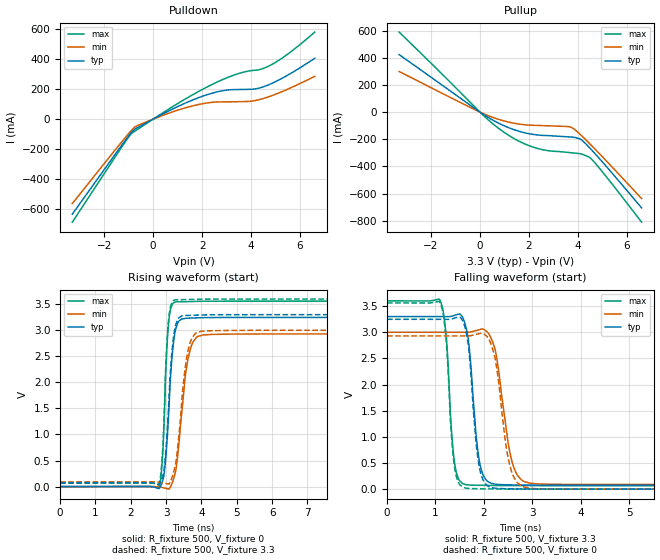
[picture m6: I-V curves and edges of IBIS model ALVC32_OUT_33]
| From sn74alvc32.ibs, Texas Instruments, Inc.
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[Model]   ALVC32_OUT_33
Model_type  Output
Vref =   0
Rref =   500
Cref =   50p
Vmeas =   1.5
| variable   typ   min   max
C_comp   7.48pF   5.11pF   11.40pF
| C_pullup   8.30pF   5.11pF   11.40pF
| C_pulldown   6.66pF   5.16pF   9.51pF
[Temperature Range]   40   100   -40
| Ambient temperature   25   85   -40
[Voltage range]   3.3   3   3.6
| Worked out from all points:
|   slope of the pulldown table from 0 to 0.495 V, typ, clamps not added: 11.6 ohm
|   slope of the pullup table from 0 to 0.495 V, typ, clamps not added: 8.84 ohm
|   rising waveform, R_fixture 500, V_fixture 0: 20-80 % time 181ps typ, 265ps min, 127ps max; typ from 0 V to 3.25 V
|   falling waveform, R_fixture 500, V_fixture 3.3: 20-80 % time 175ps typ, 264ps min, 136ps max; typ from 3.3 V to 0.073 V
|   rising waveform, R_fixture 500, V_fixture 3.3: 20-80 % time 179ps typ, 255ps min, 126ps max; typ from 0.073 V to 3.3 V
|   falling waveform, R_fixture 500, V_fixture 0: 20-80 % time 172ps typ, 243ps min, 137ps max; typ from 3.25 V to 0 V
[Pulldown]
| ALVC32_OUT_33
|   Voltage   I(typ)   I(min)   I(max)
-3.3V     -631.7mA   -561.5mA   -685mA
-1.115V   -136.4mA   -118.3mA   -145.6mA
-910mV    -93.12mA   -79.48mA   -100.6mA
-740mV    -66.58mA   -52.27mA   -79.35mA
825mV     69.55mA    49.91mA    85.75mA
2.12V     157.8mA    105.3mA    206.7mA
2.98V     192.3mA    114.9mA    272.7mA
3.985V    198.5mA    119.1mA    321.9mA
4.4V      209.9mA    132.7mA    331.5mA
4.855V    238mA      156.6mA    363.9mA
5.605V    302.5mA    207mA      445.3mA
6.6V      404.7mA    284.5mA    578.6mA
[Pullup]
| ALVC32_OUT_33
|   Voltage   I(typ)   I(min)   I(max)
-3.3V     423.4mA    299.2mA    589.2mA
100mV     -12.23mA   -8.248mA   -17.57mA
950mV     -97.85mA   -63.56mA   -144.6mA
1.595V    -141.3mA   -88.12mA   -214.5mA
2.245V    -166.3mA   -97.73mA   -262.1mA
2.8V      -173.2mA   -101.1mA   -284.5mA
3.75V     -183.9mA   -114.4mA   -299.9mA
4.115V    -201.1mA   -168.2mA   -307.3mA
4.435V    -254.9mA   -224.6mA   -330.1mA
4.555V    -278.1mA   -246.5mA   -346.3mA
5.24V     -417.4mA   -374.9mA   -494.4mA
6.6V      -705.7mA   -637.2mA   -810.8mA
[Ramp]
| ALVC32_OUT_33
| variable   typ   min   max
dV/dt_r   1.97/1.91E-10   1.79/2.92E-10   2.16/1.30E-10
dV/dt_f   1.97/1.88E-10   1.79/2.80E-10   2.14/1.42E-10
R_load = 500
[Rising Waveform]
| ALVC32_OUT_33
R_fixture =   500
C_fixture =   0
L_fixture =   0
V_fixture =   0
V_fixture_min = 0
V_fixture_max = 0
|   Time   V(typ)   V(min)   V(max)
0s        40.4pV     4.177nV    33.01pV
2.775ns   -32.21mV   -6.385mV   -28.38mV
2.9ns     108.1mV    -19.29mV   595.4mV
3ns       639.5mV    -34.64mV   2.367V
3.07ns    1.379V     -47.95mV   3.141V
3.165ns   2.471V     57.93mV    3.482V
3.28ns    3.046V     340.7mV    3.548V
3.625ns   3.232V     2.472V     3.551V
4.07ns    3.243V     2.914V     3.558V
50ns      3.247V     2.929V     3.56V
[Falling Waveform]
| ALVC32_OUT_33
R_fixture =   500
C_fixture =   0
L_fixture =   0
V_fixture =   3.3
V_fixture_min = 3
V_fixture_max = 3.6
|   Time   V(typ)   V(min)   V(max)
0s        3.3V       3V         3.6V
1.1ns     3.3V       3V         3.602V
1.23ns    3.299V     3V         2.853V
1.405ns   3.327V     3V         444.4mV
1.715ns   2.543V     3.004V     77.48mV
2ns       238.7mV    3.053V     72.08mV
2.235ns   95.03mV    2.661V     69.23mV
2.61ns    79.34mV    440.3mV    66.86mV
3.105ns   74.26mV    100mV      66.21mV
50ns      72.86mV    89.69mV    66.1mV
[Rising Waveform]
| ALVC32_OUT_33
R_fixture =   500
C_fixture =   0
L_fixture =   0
V_fixture =   3.3
V_fixture_min = 3
V_fixture_max = 3.6
|   Time   V(typ)   V(min)   V(max)
0s        72.86mV    89.69mV    66.1mV
2.775ns   42.6mV     83.19mV    39.53mV
2.9ns     191.3mV    71.49mV    679.2mV
2.995ns   717.1mV    60.22mV    2.379V
3.065ns   1.47V      50.55mV    3.17V
3.165ns   2.592V     172.8mV    3.529V
3.28ns    3.124V     488.1mV    3.588V
3.605ns   3.285V     2.56V      3.591V
4.01ns    3.295V     2.982V     3.598V
50ns      3.3V       3V         3.6V
[Falling Waveform]
| ALVC32_OUT_33
R_fixture =   500
C_fixture =   0
L_fixture =   0
V_fixture =   0
V_fixture_min = 0
V_fixture_max = 0
|   Time   V(typ)   V(min)   V(max)
0s        3.247V     2.929V     3.56V
1.1ns     3.247V     2.929V     3.557V
1.225ns   3.247V     2.929V     2.811V
1.39ns    3.268V     2.929V     453.3mV
1.65ns    2.926V     2.93V      15.24mV
1.915ns   381.5mV    2.975V     6.973mV
2.305ns   11.65mV    2.051V     2.363mV
2.57ns    5.627mV    345mV      843.5uV
3.02ns    1.765mV    10.91mV    148.7uV
50ns      40.1pV     4.177nV    32.54pV
